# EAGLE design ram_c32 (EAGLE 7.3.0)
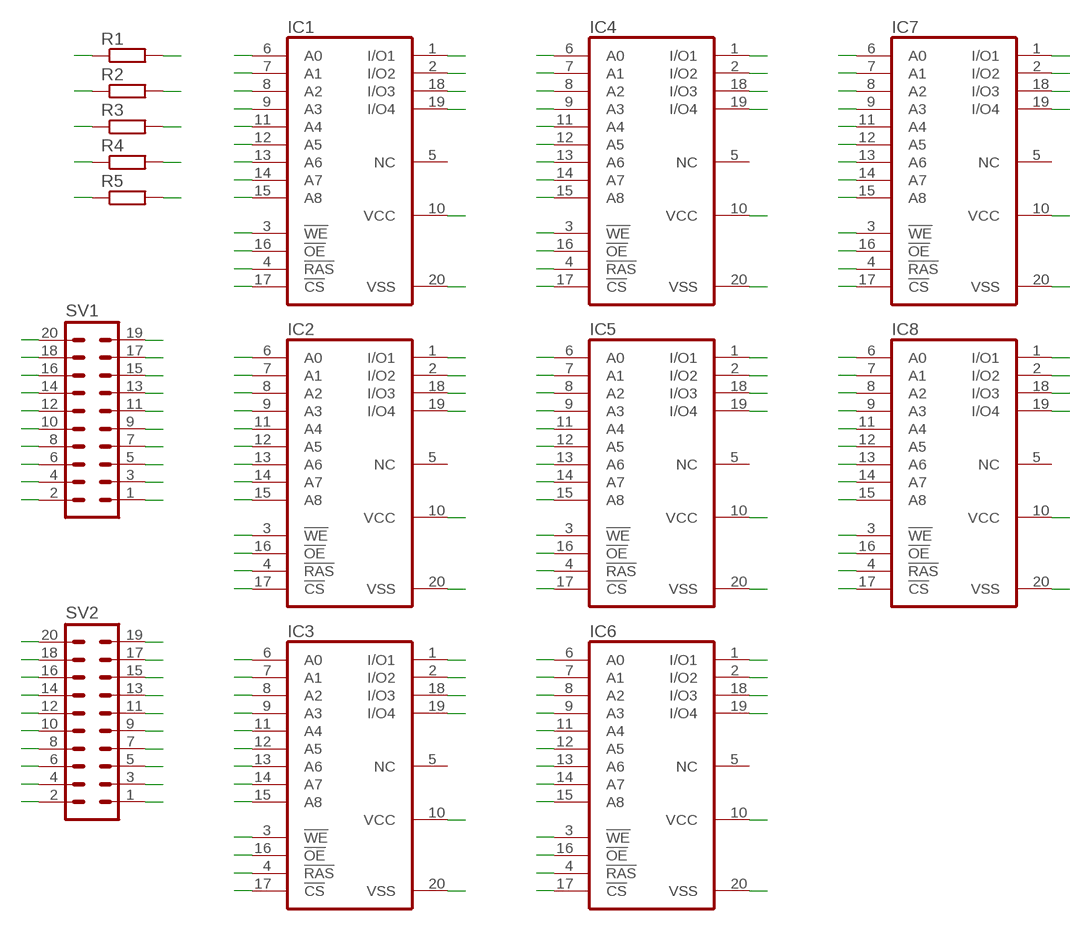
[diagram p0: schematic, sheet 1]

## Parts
IC1  514258AP  [DIL20]
IC2  514258AP  [DIL20]
IC3  514258AP  [DIL20]
IC4  514258AP  [DIL20]
IC5  514258AP  [DIL20]
IC6  514258AP  [DIL20]
IC7  514258AP  [DIL20]
IC8  514258AP  [DIL20]
R1  R-EU_M1206  [M1206]
R2  R-EU_M1206  [M1206]
R3  R-EU_M1206  [M1206]
R4  R-EU_M1206  [M1206]
R5  R-EU_M1206  [M1206]
SV1  ML20  [ML20]
SV2  ML20  [ML20]

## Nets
BEN0: IC5.16(!OE) IC6.16(!OE) IC7.16(!OE) IC8.16(!OE) R4.2
BEN0W: R4.1 SV1.10
BEN1: IC1.16(!OE) IC2.16(!OE) IC3.16(!OE) IC4.16(!OE) R5.2
BEN1W: R5.1 SV1.5
CAS0: IC5.17(!CS) IC6.17(!CS) IC7.17(!CS) IC8.17(!CS) R2.2
CAS0W: R2.1 SV1.4
CAS1: IC1.17(!CS) IC2.17(!CS) IC3.17(!CS) IC4.17(!CS) R3.2
CAS1W: R3.1 SV1.9
D0: IC1.19(I/O4) IC5.19(I/O4) SV2.20
D1: IC1.18(I/O3) IC5.18(I/O3) SV2.19
D2: IC1.2(I/O2) IC5.2(I/O2) SV2.18
D3: IC1.1(I/O1) IC5.1(I/O1) SV2.17
D4: IC2.19(I/O4) IC6.19(I/O4) SV2.16
D5: IC2.18(I/O3) IC6.18(I/O3) SV2.15
D6: IC2.2(I/O2) IC6.2(I/O2) SV2.14
D7: IC2.1(I/O1) IC6.1(I/O1) SV2.13
D8: IC3.19(I/O4) IC7.19(I/O4) SV2.12
D9: IC3.18(I/O3) IC7.18(I/O3) SV2.11
D10: IC3.2(I/O2) IC7.2(I/O2) SV2.10
D11: IC3.1(I/O1) IC7.1(I/O1) SV2.9
D12: IC4.19(I/O4) IC8.19(I/O4) SV2.8
D13: IC4.18(I/O3) IC8.18(I/O3) SV2.7
D14: IC4.2(I/O2) IC8.2(I/O2) SV2.6
D15: IC4.1(I/O1) IC8.1(I/O1) SV2.5
DRA0: IC1.6(A0) IC2.6(A0) IC3.6(A0) IC4.6(A0) IC5.6(A0) IC6.6(A0) IC7.6(A0) IC8.6(A0) SV1.20
DRA1: IC1.7(A1) IC2.7(A1) IC3.7(A1) IC4.7(A1) IC5.7(A1) IC6.7(A1) IC7.7(A1) IC8.7(A1) SV1.19
DRA2: IC1.8(A2) IC2.8(A2) IC3.8(A2) IC4.8(A2) IC5.8(A2) IC6.8(A2) IC7.8(A2) IC8.8(A2) SV1.18
DRA3: IC1.9(A3) IC2.9(A3) IC3.9(A3) IC4.9(A3) IC5.9(A3) IC6.9(A3) IC7.9(A3) IC8.9(A3) SV1.17
DRA4: IC1.11(A4) IC2.11(A4) IC3.11(A4) IC4.11(A4) IC5.11(A4) IC6.11(A4) IC7.11(A4) IC8.11(A4) SV1.16
DRA5: IC1.12(A5) IC2.12(A5) IC3.12(A5) IC4.12(A5) IC5.12(A5) IC6.12(A5) IC7.12(A5) IC8.12(A5) SV1.15
DRA6: IC1.13(A6) IC2.13(A6) IC3.13(A6) IC4.13(A6) IC5.13(A6) IC6.13(A6) IC7.13(A6) IC8.13(A6) SV1.14
DRA7: IC1.14(A7) IC2.14(A7) IC3.14(A7) IC4.14(A7) IC5.14(A7) IC6.14(A7) IC7.14(A7) IC8.14(A7) SV1.13
DRA8: IC1.15(A8) IC2.15(A8) IC3.15(A8) IC4.15(A8) IC5.15(A8) IC6.15(A8) IC7.15(A8) IC8.15(A8) SV1.12
GND: IC1.20(VSS) IC2.20(VSS) IC3.20(VSS) IC4.20(VSS) IC5.20(VSS) IC6.20(VSS) IC7.20(VSS) IC8.20(VSS) SV1.1 SV1.2 SV1.3
RAS0: IC1.4(!RAS) IC2.4(!RAS) IC3.4(!RAS) IC4.4(!RAS) IC5.4(!RAS) IC6.4(!RAS) IC7.4(!RAS) IC8.4(!RAS) R1.2
RAS0W: R1.1 SV1.11
RAS1W: SV1.6
RAS2W: SV1.7
RAS3W: SV1.8
VCC: IC1.10(VCC) IC2.10(VCC) IC3.10(VCC) IC4.10(VCC) IC5.10(VCC) IC6.10(VCC) IC7.10(VCC) IC8.10(VCC) SV2.1 SV2.2
WEH: IC3.3(!WE) IC4.3(!WE) IC7.3(!WE) IC8.3(!WE) SV2.4
WEL: IC1.3(!WE) IC2.3(!WE) IC5.3(!WE) IC6.3(!WE) SV2.3
Unconnected: IC1.5(NC) IC2.5(NC) IC3.5(NC) IC4.5(NC) IC5.5(NC) IC6.5(NC) IC7.5(NC) IC8.5(NC)

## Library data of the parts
IC1-IC8 = memory-hitachi:514258AP: MEMORY; OC_FARNELL: unknown; OC_NEWARK: unknown
R1-R5 = resistor:R-EU_: RESISTOR, European symbol
SV1 SV2 = con-atari:ML20: HARTING; OC_FARNELL: unknown; OC_NEWARK: unknown

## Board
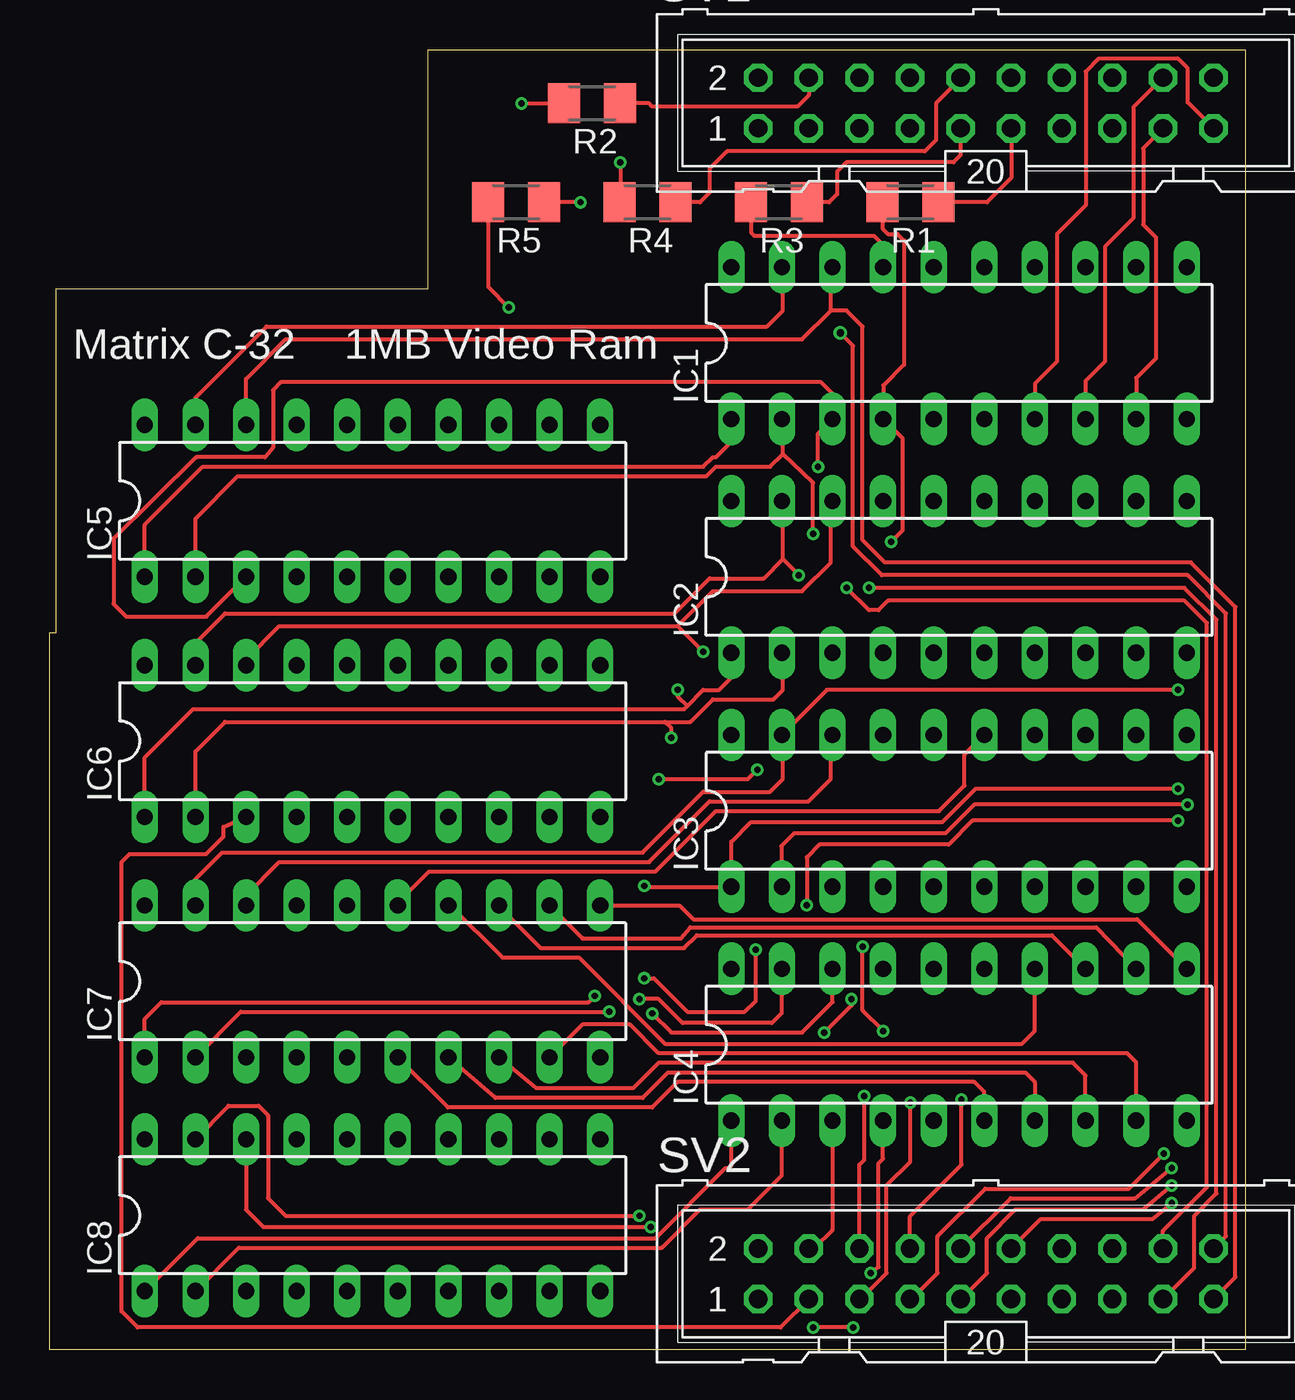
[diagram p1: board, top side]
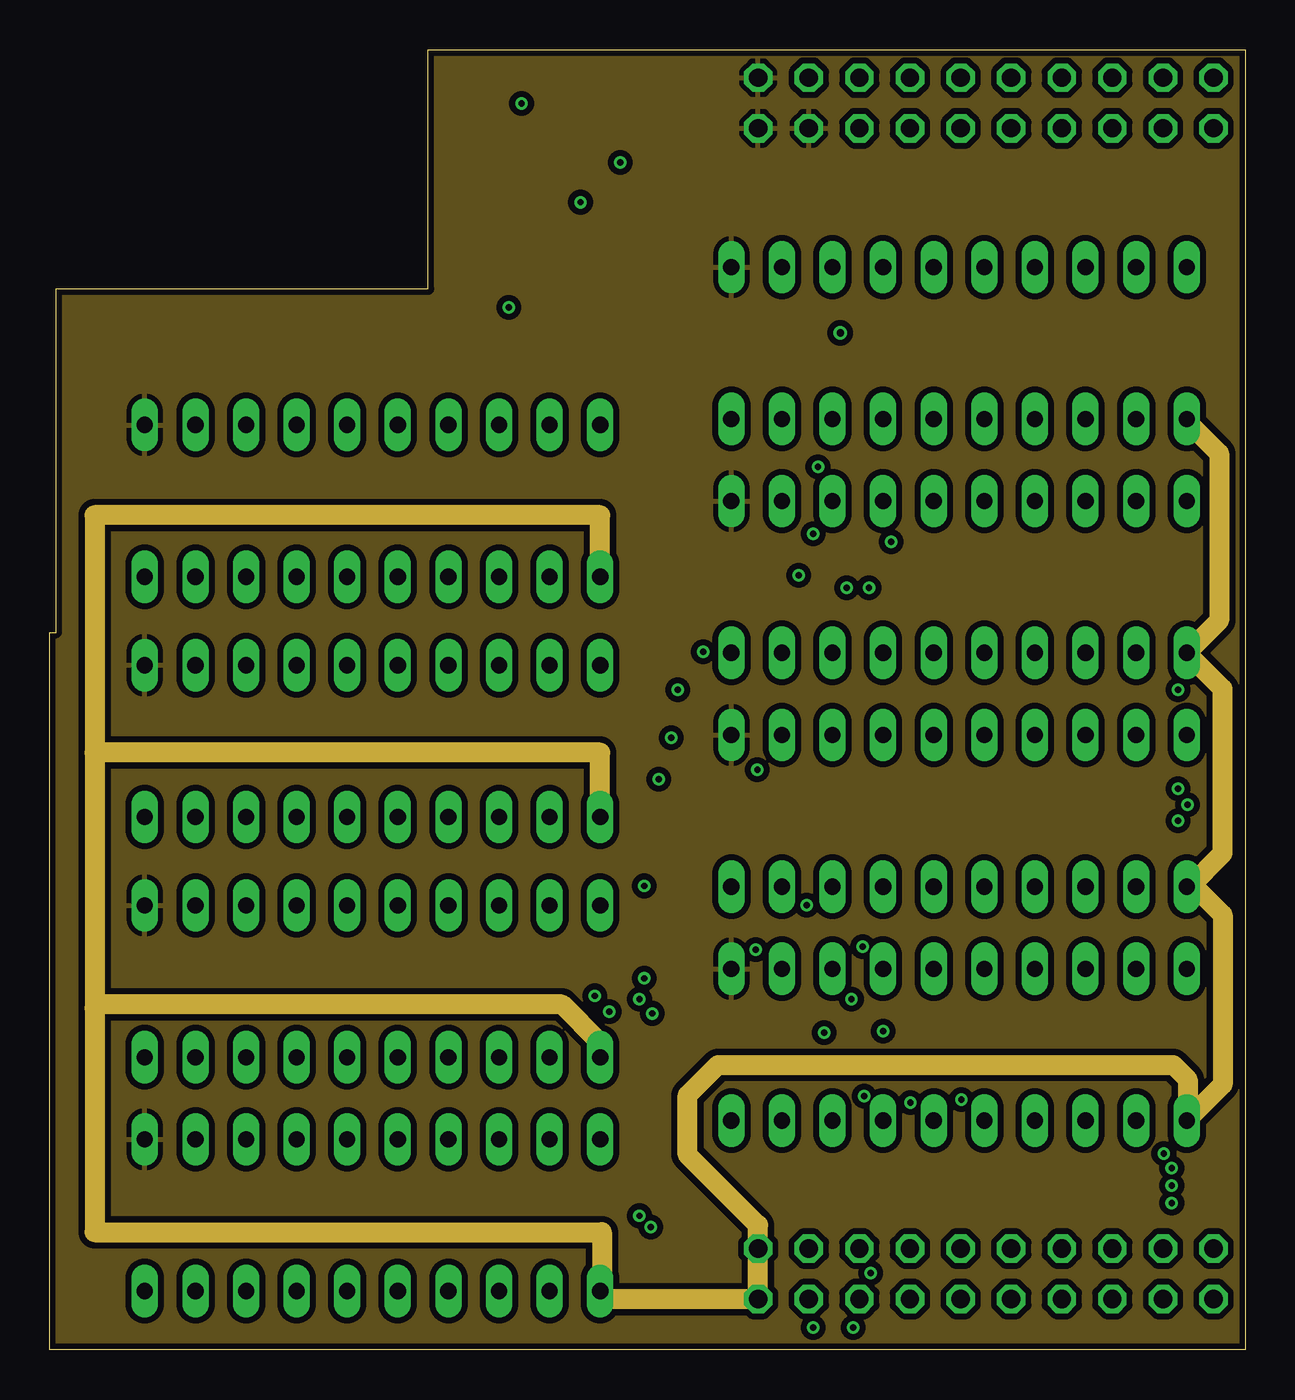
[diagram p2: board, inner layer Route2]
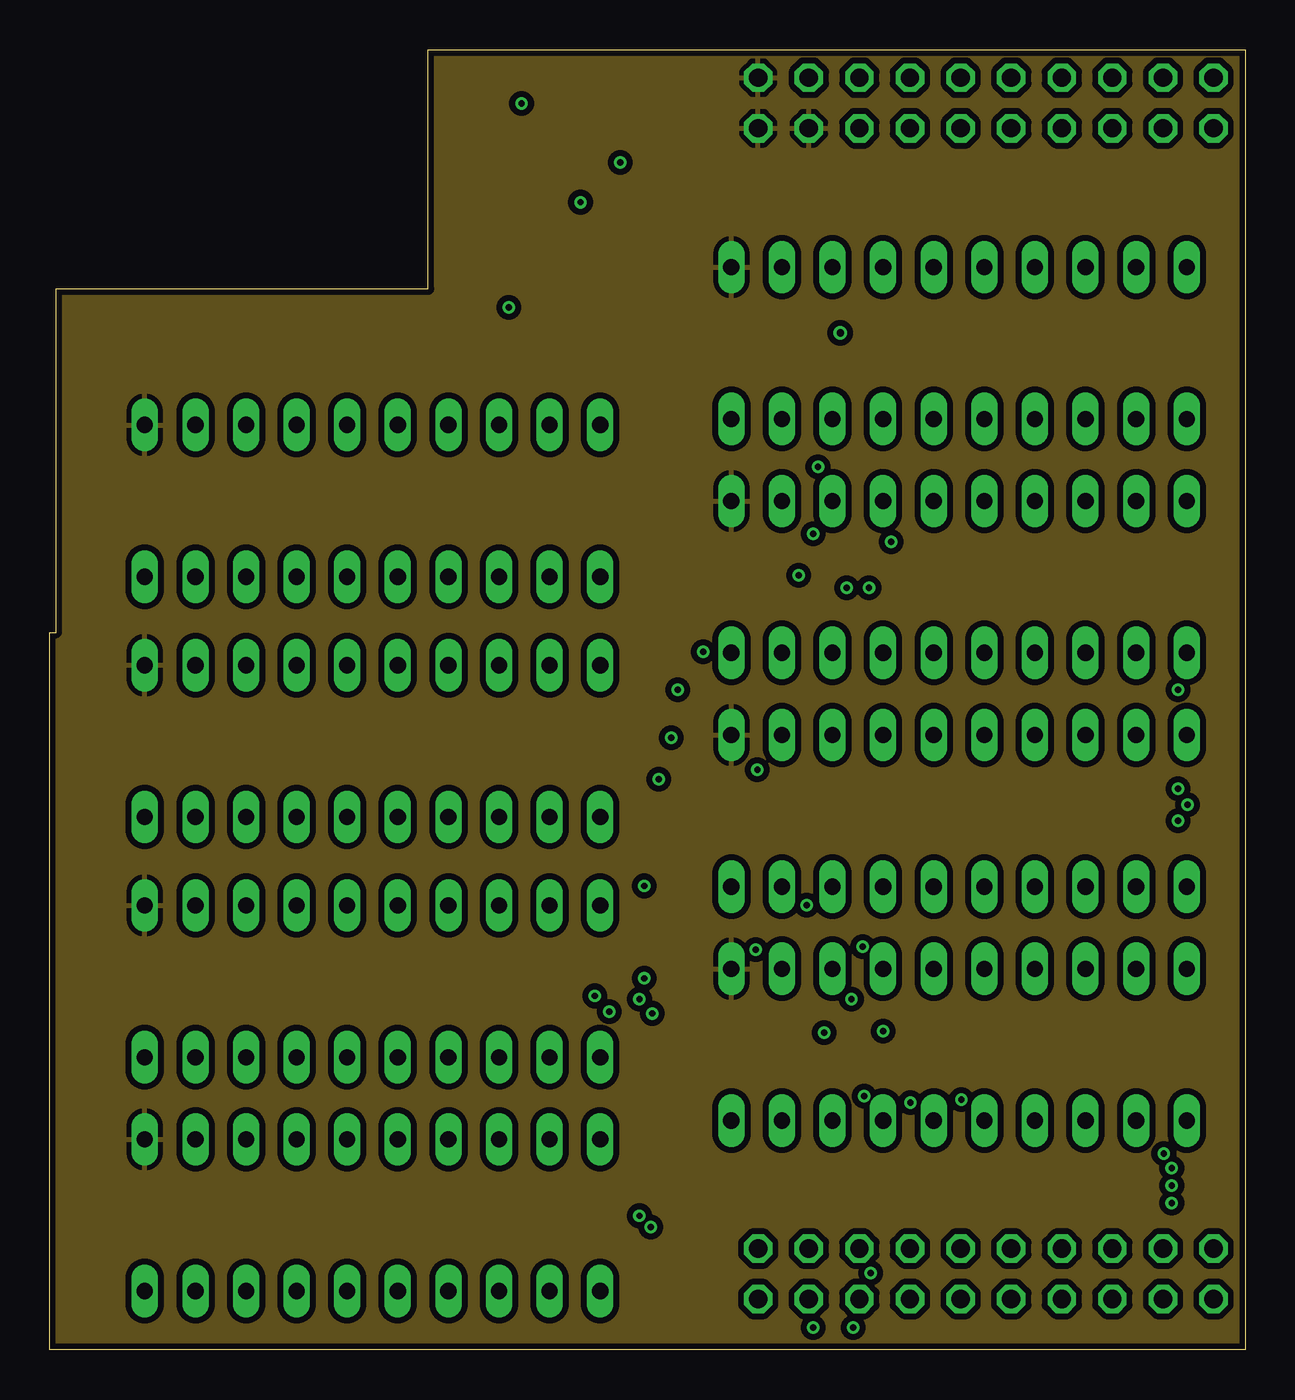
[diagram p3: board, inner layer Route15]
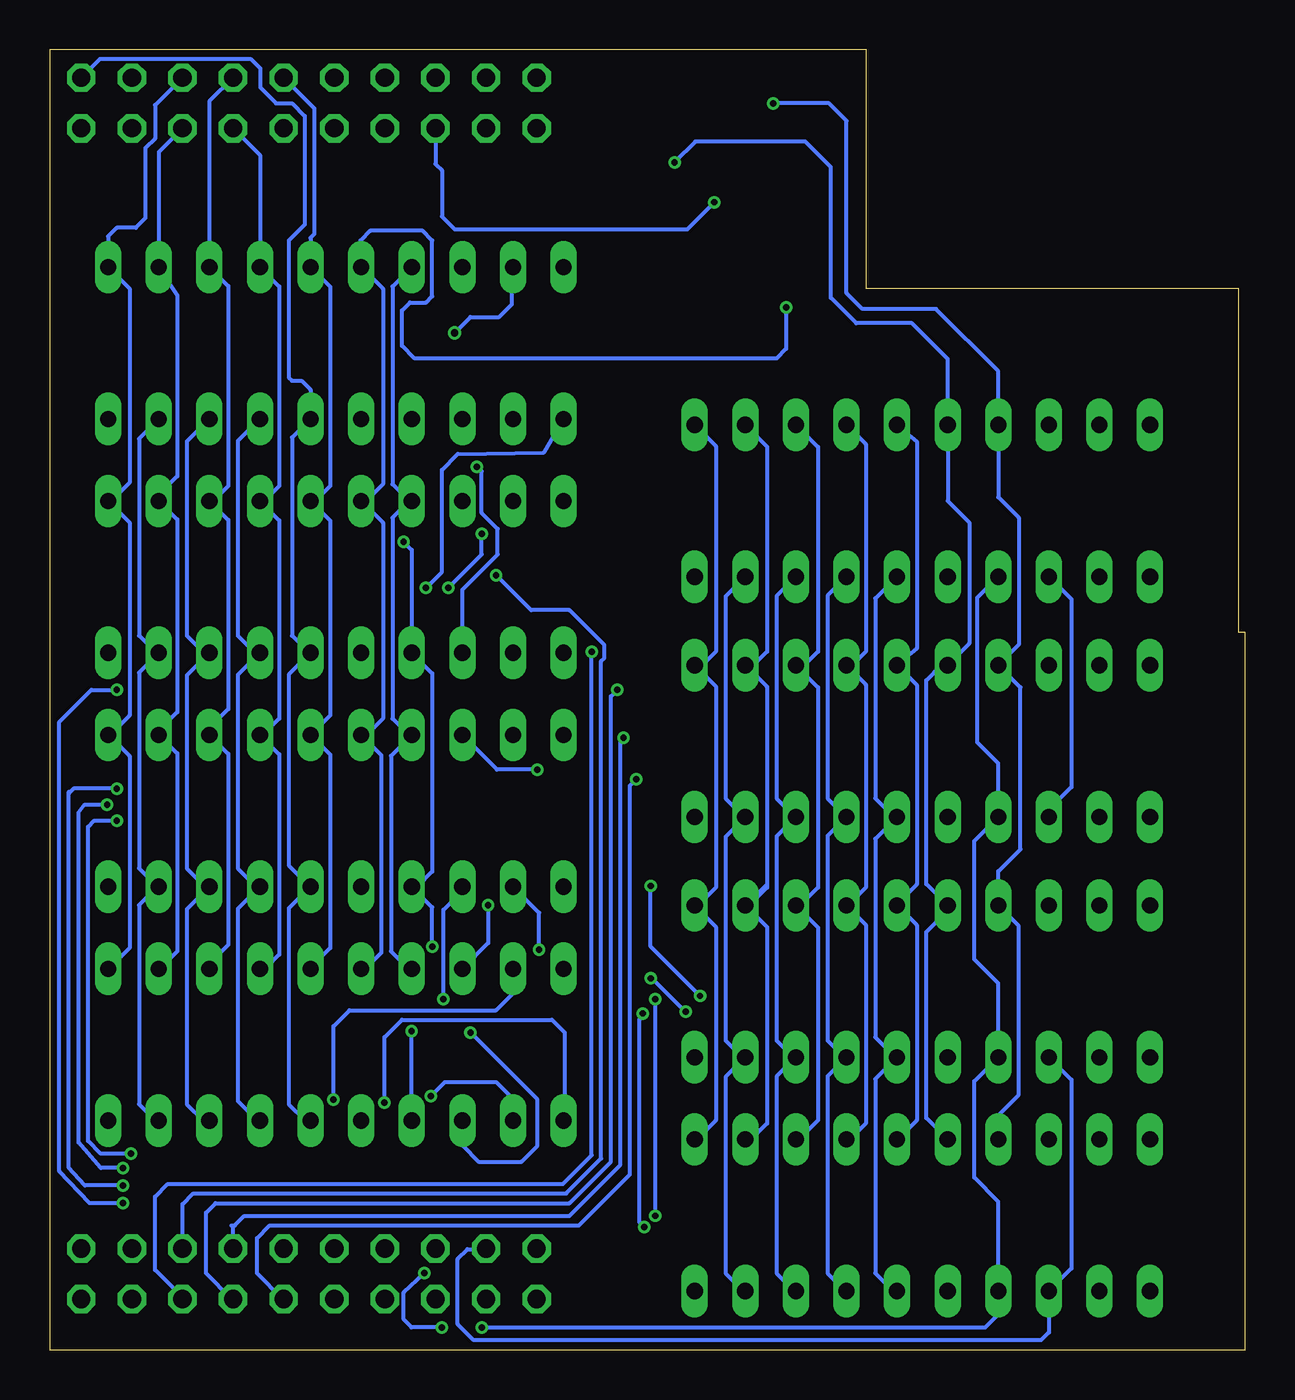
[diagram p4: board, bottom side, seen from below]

Size 60 x 65.25 mm. Coordinates in mm from the lower left corner, seen from the top.
Outline: 0,0 0,36 0.32,36 0.32,53.25 19,53.25 19,65.25 60,65.25 60,0 0,0
Copper layers (1*2+15*16): Top 0.035mm / dielectric 1.5mm / Route2 0.0175mm / dielectric 1.1mm / Route15 0.0175mm / dielectric 0.2mm / Bottom 0.035mm
Design rules "default *": minimum track width 5mil, minimum drill 12mil, track to track 5mil, track to pad 5mil, pad to pad 5mil, via to via 5mil, smd to smd 0mil, copper to edge 10mil, drill to drill 10mil, minimum pad ring 10mil, minimum via ring 6mil, stop-mask expansion 2mil, vias tented up to drill 25mil, thermal gap 10mil

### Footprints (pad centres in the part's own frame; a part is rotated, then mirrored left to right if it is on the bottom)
DIL20 = drill 0.813 long: 1 -11.43,-3.81; 2 -8.89,-3.81; 3 -6.35,-3.81; 4 -3.81,-3.81; 5 -1.27,-3.81; 6 1.27,-3.81; 7 3.81,-3.81; 8 6.35,-3.81; 9 8.89,-3.81; 10 11.43,-3.81; 11 11.43,3.81; 12 8.89,3.81; 13 6.35,3.81; 14 3.81,3.81; 15 1.27,3.81; 16 -1.27,3.81; 17 -3.81,3.81; 18 -6.35,3.81; 19 -8.89,3.81; 20 -11.43,3.81
M1206 = smd 1.6 x 2: 1 -1.4,0; 2 1.4,0
ML20 = drill 0.914 octagon: 1 -11.43,-1.27; 2 -11.43,1.27; 3 -8.89,-1.27; 4 -8.89,1.27; 5 -6.35,-1.27; 6 -6.35,1.27; 7 -3.81,-1.27; 8 -3.81,1.27; 9 -1.27,-1.27; 10 -1.27,1.27; 11 1.27,-1.27; 12 1.27,1.27; 13 3.81,-1.27; 14 3.81,1.27; 15 6.35,-1.27; 16 6.35,1.27; 17 8.89,-1.27; 18 8.89,1.27; 19 11.43,-1.27; 20 11.43,1.27

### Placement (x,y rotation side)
IC1  45.64,50.53 0 top
IC2  45.64,38.79 0 top
IC3  45.64,27.05 0 top
IC4  45.64,15.31 0 top
IC5  16.2,42.61 0 top
IC6  16.2,30.55 0 top
IC7  16.2,18.49 0 top
IC8  16.2,6.75 0 top
R1  43.2,57.6 180 top
R2  27.22,62.57 180 top
R3  36.6,57.6 180 top
R4  30,57.6 180 top
R5  23.4,57.6 180 top
SV1  46.99,62.58 0 top
SV2  46.99,3.81 0 top

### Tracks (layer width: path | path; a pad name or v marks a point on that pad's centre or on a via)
BEN0  (via drill 0.32)
  Top 0.2: v28.64,59.6 28.64,57.64 R4.2
  Bottom 0.2: v28.64,59.6 27.6,60.64 22.08,60.64 20.8,59.36 20.8,52.8 19.52,51.52 16.72,51.52 14.93,49.73 IC5.16 14.93,42.61 13.84,41.52 13.84,35.45 IC6.16 15.24,34.36 16,33.6 16,23.37 IC7.16 14.93,22.03 16,20.96 16,11.63 IC8.16
BEN0W
  Top 0.2: SV1.10 45.72,63.8 44.48,62.56 44.48,60.72 43.92,60.16 34,60.16 33.12,59.28 33.12,58.08 32.64,57.6 R4.1
BEN1  (via drill 0.32)
  Top 0.2: R5.2 22,53.36 v23.04,52.32
  Bottom 0.2: IC4.16 44.16,19.12 43.36,19.92 43.36,29.85 IC3.16 44.1,30.86 43.28,31.68 43.28,41.51 IC2.16 44.12,42.6 43.28,43.44 43.28,53.25 IC1.16 44.4,54.37 44.4,55.68 43.92,56.16 41.28,56.16 40.8,55.68 40.8,52.88 41.12,52.56 41.92,52.56 42.32,52.16 42.32,50.4 41.68,49.76 23.52,49.76 23.04,50.24 v23.04,52.32
BEN1W  (via drill 0.32)
  Top 0.2: v26.64,57.6 R5.1
  Bottom 0.2: SV1.5 40.64,59.52 40.32,59.2 40.32,56.88 39.68,56.24 28,56.24 v26.64,57.6
CAS0  (via drill 0.32)
  Top 0.2: v23.68,62.56 R2.2
  Bottom 0.2: v23.68,62.56 20.88,62.56 20,61.68 20,53.04 19.2,52.24 15.52,52.24 12.39,49.11 IC5.17 12.39,42.79 11.36,41.76 11.36,35.39 IC6.17 11.28,33.25 11.28,25.12 12.39,24.01 IC7.17 11.36,21.27 11.36,12.8 12.39,11.77 IC8.17
CAS0W
  Top 0.2: SV1.4 38.1,62.98 37.52,62.4 30.24,62.4 30.08,62.56 R2.1
CAS1
  Top 0.2: R3.2 35.2,56.08 35.36,55.92 41.36,55.92 41.84,55.44 IC1.17
  Bottom 0.2: IC1.17 42.8,53.37 42.8,43.44 41.96,42.6 | 41.96,42.6 IC2.17 | 41.96,42.6 42.8,41.76 42.8,31.68 41.98,30.86 IC3.17 42.88,29.81 42.88,20 42,19.12 IC4.17
CAS1W
  Top 0.2: SV1.9 45.72,59.96 45.36,59.6 40,59.6 39.52,59.12 39.52,58 39.12,57.6 R3.1
D0  (via drill 0.36)
  Top 0.2: IC5.19 7.31,47.79 10.88,51.36 36,51.36 36.8,52.16 36.8,54.29 IC1.19 | SV2.20 59.04,5.7 59.04,36.96 57.12,38.88 41.76,38.88 40.32,40.32 40.32,50.4 v39.68,51.04
  Bottom 0.2: v39.68,51.04 38.88,51.84 37.44,51.84 36.8,52.48 36.8,53.76 36.75,53.81 IC1.19
D1
  Top 0.2: IC5.18 9.85,48.73 11.84,50.72 37.76,50.72 39.2,52.16 | 39.2,52.16 39.2,54.25 IC1.18 | SV2.19 59.52,3.64 59.52,37.28 57.28,39.52 41.92,39.52 40.8,40.64 40.8,51.36 40,52.16 39.2,52.16
D2  (via drill 0.32)
  Top 0.2: IC5.2 7.31,41.71 9.44,43.84 32.96,43.84 33.44,44.32 36.16,44.32 36.8,44.96 | 36.8,44.96 36.8,46.67 IC1.2 | SV2.18 55.88,5.96 58.08,8.16 58.08,36.48 56.96,37.6 42.08,37.6 41.6,37.12 41.12,37.12 v40,38.24 | v38.32,40.96 38.32,43.52 36.8,44.96
  Bottom 0.2: v40,38.24 38.32,39.92 v38.32,40.96
D3  (via drill 0.32)
  Top 0.2: IC5.1 4.77,41.41 7.68,44.32 32.8,44.32 33.28,44.8 33.44,44.8 34.08,45.44 34.08,46.59 IC1.1 | SV2.17 57.44,4.1 57.44,6.72 58.56,7.84 58.56,36.64 56.96,38.24 v41.12,38.24
  Bottom 0.2: v41.12,38.24 40.32,39.04 40.32,44.16 39.52,44.96 35.2,45.04 35.17,45.07 IC1.1
D4  (via drill 0.32)
  Top 0.2: IC6.19 7.31,35.47 8.8,36.96 31.36,36.96 33.12,38.72 35.84,38.72 36.8,39.68 | 36.8,39.68 36.8,42.55 IC2.19 | v37.6,38.88 36.8,39.68
  Bottom 0.2: SV2.16 53.34,7.3 52.8,7.84 34.08,7.84 32.32,9.6 32.32,34.56 32.16,34.72 32.16,35.36 33.92,37.12 35.84,37.12 v37.6,38.88
D5  (via drill 0.32)
  Top 0.2: IC6.18 9.85,34.65 11.52,36.32 31.52,36.32 | 31.52,36.32 33.28,38.08 37.76,38.08 39.2,39.52 39.2,42.51 IC2.18 | v32.8,35.04 31.52,36.32
  Bottom 0.2: SV2.15 53.34,2.62 54.72,4 54.72,7.68 54.08,8.32 34.24,8.32 32.8,9.76 v32.8,35.04
D6  (via drill 0.32)
  Top 0.2: IC6.2 7.31,30.03 8.8,31.52 30.88,31.52 | 30.88,31.52 32.16,31.52 33.28,32.64 36.32,32.64 36.8,33.12 36.8,34.93 IC2.2 | v31.2,30.72 31.2,31.2 30.88,31.52
  Bottom 0.2: SV2.14 50.8,6.16 50.88,6.24 50.72,6.24 50.24,6.72 33.92,6.72 31.36,9.28 31.36,30.56 v31.2,30.72
D7  (via drill 0.32)
  Top 0.2: IC6.1 4.77,29.73 7.2,32.16 31.84,32.16 32,32.32 | 32,32.32 32.8,33.12 33.6,33.12 34.24,33.76 34.24,34.95 IC2.1 | v31.52,33.12 31.52,32.8 32,32.32
  Bottom 0.2: SV2.13 50.86,2.54 52.16,3.84 52.16,6.88 51.68,7.36 33.92,7.36 31.84,9.44 31.84,32.8 v31.52,33.12
D8  (via drill 0.32)
  Top 0.2: IC7.19 7.31,23.63 8.64,24.96 29.76,24.96 32.8,28 36.16,28 36.8,28.64 36.8,30.81 IC3.19 39.01,33.12 v56.64,33.12 | SV2.12 48.28,5.08 49.76,6.56 55.36,6.56 v56.32,7.36
  Bottom 0.2: v56.32,7.36 58,7.36 59.52,8.96 59.52,31.52 57.92,33.12 v56.64,33.12
D9  (via drill 0.32)
  Top 0.2: IC7.18 9.85,22.81 11.52,24.48 30.08,24.48 33.12,27.52 38.08,27.52 39.2,28.64 39.2,30.77 IC3.18 | v30.56,28.64 35.04,28.64 v35.52,29.12
  Bottom 0.2: SV2.11 48.3,2.54 49.6,3.84 49.6,5.6 48.96,6.24 33.44,6.24 30.88,8.8 30.88,28.32 v30.56,28.64 | v35.52,29.12 37.55,29.12 IC3.18
D10  (via drill 0.32)
  Top 0.2: SV2.10 48.24,7.6 54.48,7.6 v56.32,9.12 | v57.12,27.36 46.4,27.36 44.96,25.92 37.36,25.92 36.72,25.28 36.72,23.27 IC3.2 | IC7.2 9.59,16.96 v28.08,16.96 | v29.84,18.64 30.32,18.64 32,16.96 34.88,16.96 35.44,17.52 v35.44,20.08
  Bottom 0.2: v56.32,9.12 57.44,9.12 58.56,10.4 58.56,26.96 58.24,27.36 v57.12,27.36 | v28.08,16.96 29.76,18.64 v29.84,18.64 | v35.44,20.08 35.44,21.93 IC3.2
D11  (via drill 0.32)
  Top 0.2: SV2.9 45.74,2.54 47.04,3.84 47.04,5.6 48.48,7.04 54.88,7.04 v56.32,8.24 | v56.64,28.16 46.48,28.16 44.8,26.48 35.2,26.48 34.21,25.49 IC3.1 29.88,23.24 v29.84,23.28 | IC7.1 4.77,16.61 5.6,17.44 27.04,17.44 v27.36,17.76
  Bottom 0.2: v56.32,8.24 58.24,8.24 59.04,9.12 59.04,27.92 | 59.04,27.92 59.04,28 | v56.64,28.16 58.8,28.16 59.04,27.92 | v27.36,17.76 29.84,20.24 v29.84,23.28
D12  (via drill 0.32)
  Top 0.2: SV2.8 43.18,6.7 45.76,9.28 v45.76,12.56 | IC8.19 8.96,12.21 8.96,12.24 10.48,12.24 10.96,11.76 10.96,7.6 11.84,6.72 v29.6,6.72 | IC4.19 36.75,16.91 36.24,16.4 31.76,16.4 30.56,17.6 v29.6,17.6
  Bottom 0.2: v45.76,12.56 45.76,16.24 44.96,17.04 37.6,17.04 36.8,17.84 36.8,19.07 IC4.19 | v29.6,6.72 v29.6,17.6
D13  (via drill 0.32)
  Top 0.2: SV2.7 43.26,2.54 44.56,3.84 44.56,5.68 46.96,8.08 54.16,8.08 v55.92,9.84 | v56.64,26.56 46.32,26.56 45.12,25.36 38.64,25.36 38,24.72 v38,22.32 | IC8.18 9.85,7.03 10.72,6.16 v30.16,6.16 | v30.24,16.88 31.2,15.92 37.76,15.92 39.29,17.45 IC4.18
  Bottom 0.2: v55.92,9.84 57.44,9.84 58.08,10.48 58.08,26.24 57.76,26.56 v56.64,26.56 | v38,22.32 38,20.41 IC4.18 | v30.16,6.16 30.4,6.4 30.4,16.56 30.24,16.72 v30.24,16.88
D14  (via drill 0.32)
  Top 0.2: IC8.2 9.49,5.12 30.72,5.12 32.64,7.04 35.04,7.04 36.75,8.75 IC4.2 | SV2.6 40.64,9.28 40.88,9.52 v40.88,12.72
  Bottom 0.2: v40.88,12.72 40.16,13.44 37.6,13.44 36.75,12.59 IC4.2
D15  (via drill 0.32)
  Top 0.2: IC8.1 7.43,5.6 30.4,5.6 33.92,9.12 34.08,9.12 34.21,9.25 IC4.1 | SV2.5 40.7,2.54 42,3.84 42,8.24 43.2,9.44 v43.2,12.4
  Bottom 0.2: v43.2,12.4 43.2,15.68 42.32,16.56 34.8,16.56 34.16,15.92 34.16,11.55 IC4.1
DRA0
  Top 0.2: IC4.6 46.91,12.93 46.4,13.44 31.52,13.44 30.24,12.16 19.99,12.16 IC7.6
  Bottom 0.2: SV1.20 57.47,64.8 49.92,64.8 49.44,64.32 49.44,63.36 48.64,62.56 47.84,62.56 47.2,61.92 47.2,56.48 48,55.68 48,48.8 47.84,48.64 47.36,48.64 46.91,48.19 IC1.6 47.84,45.79 47.84,35.84 46.98,34.98 IC2.6 48,33.89 48,24.32 IC3.6 | IC5.6 18.56,37.71 18.56,27.68 17.62,26.74 IC6.6 18.56,25.65 18.56,15.68 17.56,14.68 IC7.6 18.56,13.59 18.56,3.84 17.66,2.94 IC8.6 | IC3.6 | IC3.6 48,22.16 48,12.32 47.18,11.5 IC4.6
DRA1
  Top 0.2: SV1.19 57.12,62.61 57.12,64.32 56.64,64.8 52.64,64.8 52,64.16 52,57.44 50.56,56 50.56,49.6 49.45,48.49 IC1.7 | IC7.7 22.37,12.64 29.76,12.64 31.04,13.92 48.96,13.92 49.44,13.44 IC4.7
  Bottom 0.2: IC5.7 20.96,37.85 20.96,27.68 IC6.7 20.96,25.79 20.96,15.52 20.12,14.68 IC7.7 20.96,13.73 20.96,3.84 20.06,2.94 IC8.7 | IC1.7 50.56,45.61 50.56,35.84 49.7,34.98 IC2.7 50.56,33.87 50.56,24.16 49.64,23.24 IC3.7 50.56,22.13 50.56,12.48 49.58,11.5 IC4.7
DRA2
  Top 0.2: SV1.18 54.4,62.37 54.4,56.8 52.96,55.36 52.96,49.6 51.99,48.63 IC1.8 | IC7.8 24.43,13.12 29.28,13.12 30.56,14.4 51.36,14.4 51.99,13.77 IC4.8
  Bottom 0.2: IC5.8 23.52,37.83 23.52,27.68 22.58,26.74 IC6.8 23.52,25.77 23.52,15.52 22.68,14.68 IC7.8 23.52,13.71 23.52,3.84 22.62,2.94 IC8.8 | IC1.8 53.12,45.59 53.12,35.84 52.26,34.98 IC2.8 53.12,33.85 53.12,24.16 52.2,23.24 IC3.8 53.12,22.11 53.12,12.32 52.3,11.5 IC4.8
DRA3
  Top 0.2: SV1.17 54.88,60.31 54.88,56.48 55.52,55.84 55.52,49.76 54.53,48.77 IC1.9 | IC7.9 26.73,16.32 29.12,16.32 30.56,14.88 54.08,14.88 54.53,14.43 IC4.9
  Bottom 0.2: IC5.9 26.08,37.81 26.08,27.68 25.14,26.74 IC6.9 26.08,25.75 26.08,15.52 25.24,14.68 IC7.9 26.08,13.69 26.08,3.84 25.18,2.94 IC8.9 | IC1.9 55.52,45.73 55.52,35.84 54.66,34.98 IC2.9 55.52,33.99 55.52,24.16 54.6,23.24 | 54.6,23.24 IC3.9 | 54.6,23.24 55.52,22.32 55.52,12.32 54.7,11.5 IC4.9
DRA4
  Top 0.2: IC7.11 31.62,22.3 32.32,21.6 54.59,21.6 IC4.11
  Bottom 0.2: SV1.16 54.72,62.47 54.72,60.8 55.2,60.32 55.2,56.8 55.68,56.32 56.64,56.32 57.07,55.89 IC1.11 56,53.27 56,43.52 56.92,42.6 IC2.11 56,41.53 56,31.84 56.98,30.86 IC3.11 56,29.79 56,20.16 57.04,19.12 IC4.11 | IC5.11 26.56,45.35 26.56,35.04 27.24,34.36 IC6.11 26.56,33.29 26.56,23.2 27.46,22.3 IC7.11 26.56,21.23 26.56,11.52 27.52,10.56 IC8.11
DRA5
  Top 0.2: IC4.12 52.53,21.2 32.16,21.2 31.68,20.64 26.72,20.64 26.72,20.67 IC7.12
  Bottom 0.2: SV1.15 54.53,60.12 IC1.12 53.6,52.93 53.6,43.84 54.53,42.91 IC2.12 53.6,41.67 53.6,32 54.53,31.07 IC3.12 53.6,29.93 53.6,20 54.48,19.12 IC4.12 | IC5.12 24,45.33 24,35.04 24.68,34.36 IC6.12 | IC6.12 24.01,33.28 24,33.28 | 24,23.36 24,23.2 24.9,22.3 IC7.12 24,21.21 24,11.36 24.8,10.56 IC8.12 | IC6.12 24,33.28 | 24,33.28 24,23.36 | 24,23.36 25.12,22.24
DRA6
  Top 0.2: IC7.13 22.55,22.25 24.64,20.16 31.84,20.16 32.48,20.8 50.31,20.8 IC4.13
  Bottom 0.2: SV1.14 51.99,62.66 IC1.13 51.04,53.39 51.04,43.36 51.8,42.6 IC2.13 51.04,41.65 51.04,32.16 51.99,31.21 IC3.13 51.04,29.91 51.04,20.32 51.99,19.37 IC4.13 | IC5.13 21.44,45.31 21.44,35.04 22.12,34.36 IC6.13 21.44,33.25 21.44,23.2 22.34,22.3 IC7.13 21.44,21.19 21.44,11.52 22.4,10.56 IC8.13
DRA7
  Top 0.2: IC7.14 20.1,22.3 22.72,19.68 26.56,19.68 30.88,15.36 48.8,15.36 49.44,16 IC4.14
  Bottom 0.2: SV1.13 49.45,59.96 IC1.14 48.48,53.37 48.48,43.36 49.24,42.6 IC2.14 48.48,41.63 48.48,31.68 49.3,30.86 IC3.14 48.48,29.89 48.48,19.84 49.2,19.12 IC4.14 | IC5.14 19.04,45.45 19.04,35.04 19.72,34.36 IC6.14 19.04,33.39 19.04,23.2 19.94,22.3 IC7.14 19.04,21.33 19.04,11.36 19.84,10.56 IC8.14
DRA8
  Top 0.2: IC3.15 45.92,29.87 45.92,28.32 44.64,27.04 33.44,27.04 30.4,24 19.04,24 17.47,22.43 IC7.15
  Bottom 0.2: SV1.12 46.72,62.31 46.72,56 46.91,55.81 IC1.15 45.92,53.35 45.92,43.36 46.68,42.6 IC2.15 45.92,41.61 45.92,31.84 IC3.15 45.92,29.87 45.92,20.16 46.91,19.17 IC4.15 | IC5.15 16.48,45.59 16.48,35.2 IC6.15 16.48,33.37 16.48,23.36 17.47,22.37 IC7.15 16.48,21.31 16.48,11.52 17.44,10.56 IC8.15
GND
  pour Route2 (isolate 0.305): 19.04,65 60,65 60,-0.08 0,-0.08 0,36 0.32,36 0.32,53.2 19.04,53.2
  pour Route15 (isolate 0.305): 19.08,65.17 60.03,65.17 60.03,-0.06 0.06,-0.06 0.06,35.99 0.36,35.99 0.36,53.26 19.08,53.26 19.08,65.11
RAS0  (via drill 0.32)
  Top 0.2: v40.32,1.12 v38.32,1.12 | v41.2,3.84 41.6,4.16 41.6,9.36 41.83,9.59 IC4.4 | v41.84,16 40.8,17.04 v40.8,20.24 | v42.24,40.56 42.8,41.12 42.8,45.75 IC1.4 41.84,48.4 42.88,49.44 42.88,55.68 42.56,56 42.08,56 41.8,56.28 R1.2
  Bottom 0.2: v38.32,1.12 13.04,1.12 12.4,1.76 IC8.4 12.39,7.43 13.6,8.64 13.6,13.47 IC7.4 12.39,18.39 13.6,19.6 13.6,25.53 IC6.4 12.39,29.43 13.44,30.48 13.44,37.75 IC5.4 | v40.32,1.12 41.84,1.12 42.24,1.52 42.24,2.88 v41.2,3.84 | IC4.4 v41.84,16 | v40.8,20.24 40.8,22.21 IC3.4 41.56,23.24 40.8,24 40.8,33.95 IC2.4 41.83,40.15 v42.24,40.56
RAS0W
  Top 0.2: SV1.11 48.26,58.82 47.04,57.6 R1.1
VCC
  Route2 1.016: IC5.10 27.63,41.89 2.25,41.89 2.25,29.97 | 2.25,29.97 2.25,17.14 | 2.25,17.14 2.25,5.9 27.71,5.9 27.71,2.94 IC8.10 28.03,2.54 SV2.1 SV2.2 35.56,6.25 32.02,9.79 32.02,12.77 33.54,14.29 56.39,14.29 57.12,13.56 57.12,11.55 IC4.10 58.88,13.31 58.88,21.83 57.47,23.24 IC3.10 57.19,23.24 58.88,24.93 58.88,33.17 IC2.10 58.7,36.61 58.7,44.99 57.07,46.62 IC1.10 | IC6.10 27.63,29.97 2.25,29.97 | IC7.10 27.63,15.4 25.7,17.33 2.43,17.33 2.25,17.14
WEH  (via drill 0.32)
  Top 0.2: IC4.3 39.28,6 38.36,5.08 SV2.4 | v38.88,15.92 40.24,17.28 v40.24,17.6
  Bottom 0.2: IC7.3 8.72,13.55 8.72,4.08 IC8.3 9.85,0.87 10.24,0.48 38.72,0.48 39.52,1.28 39.52,4.56 39.04,5.04 38.14,5.04 SV2.4 | IC4.3 39.29,10.25 38.48,9.44 36.32,9.44 35.52,10.24 35.52,12.56 v38.88,15.92 | v40.24,17.6 40.24,22.08 39.29,23.03 IC3.3
WEL  (via drill 0.32)
  Top 0.2: IC5.3 7.85,36.8 3.84,36.8 3.2,37.44 3.2,40.72 7.36,44.8 10.8,44.8 11.2,45.28 11.2,48.16 11.6,48.56 38.72,48.56 39.29,47.99 IC1.3 38.56,45.99 v38.56,44.32 | SV2.3 36.68,1.12 4.4,1.12 3.6,1.92 3.6,24.48 4,24.88 7.84,24.88 8.72,25.76 8.72,26.24 IC6.3
  Bottom 0.2: IC5.3 8.72,37.67 8.72,28.24 9.85,27.11 IC6.3 | IC2.3 39.29,38.15 37.52,39.92 37.52,41.2 38.32,42 38.32,44.08 v38.56,44.32

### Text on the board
tNames: Matrix C-32 1MB Video Ram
